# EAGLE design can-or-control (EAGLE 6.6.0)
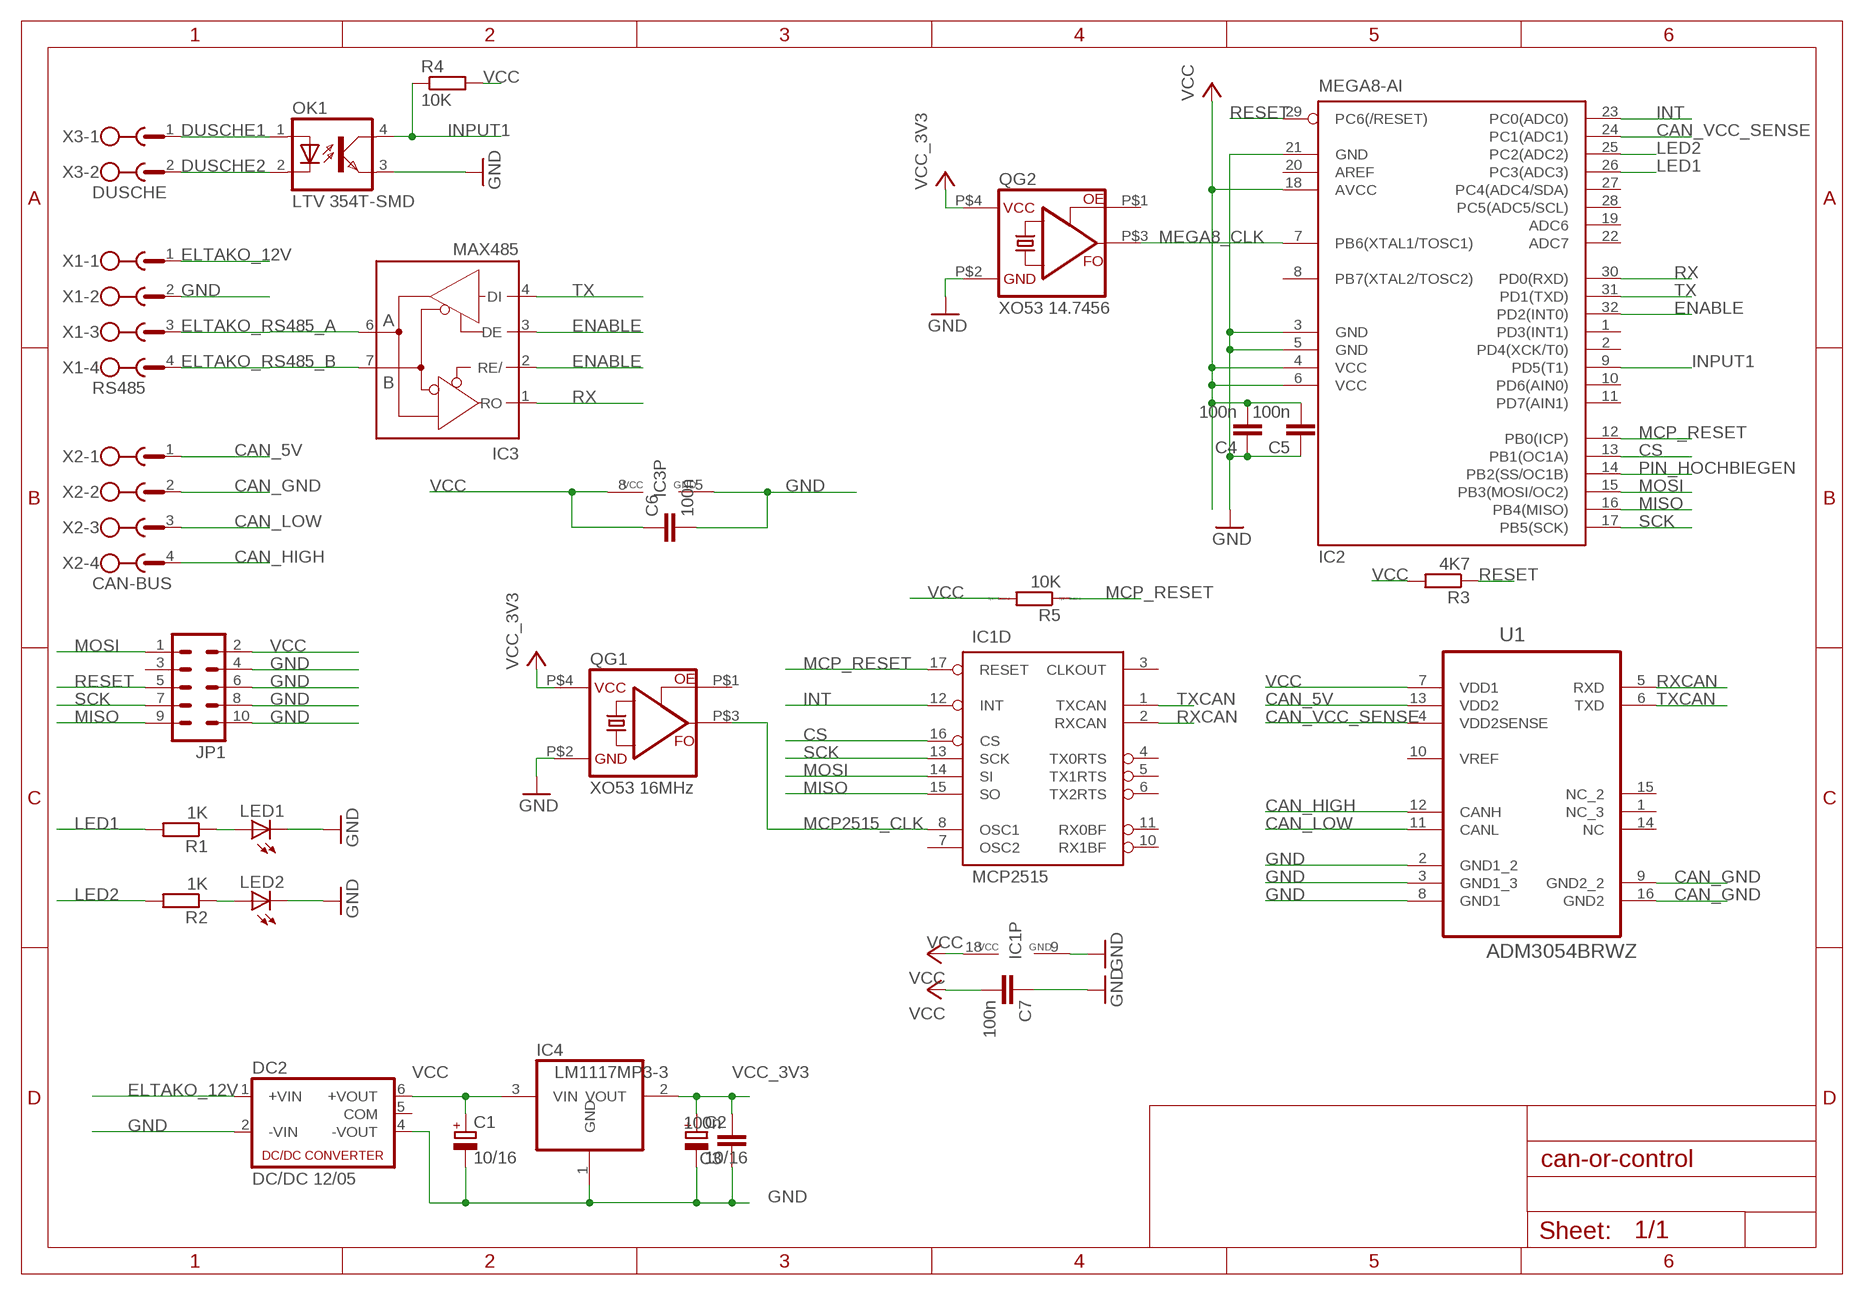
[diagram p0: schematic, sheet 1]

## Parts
C1  10/16  CPOL-EUSMCA  [SMC_A]
C2  10/16  CPOL-EUSMCA  [SMC_A]
C3  100n  C-EUC0805  [C0805]
C4  100n  C-EUC0805  [C0805]
C5  100n  C-EUC0805  [C0805]
C6  100n  C-EUC0805  [C0805]
C7  100n  C-EUC0805  [C0805]
DC2  DC/DC 12/05  NMA  [NMA]
IC1  MCP2515  MCP2515SO  [SO-18W]
IC2  MEGA8-AI  [TQFP32-08]
IC3  MAX485  MAX481CSA  [SO08]
IC4  LM1117MP3-3  REG1117  [SOT223]
JP1  ML10  [ML10]
LED1  LED3MM  [LED3MM]
LED2  LED3MM  [LED3MM]
OK1  LTV 354T-SMD  LTV816S  [SMD4]
QG1  XO53 16MHz  CRYSTALRESONATORXO53  [XO53]
QG2  XO53 14.7456  CRYSTALRESONATORXO53  [XO53]
R1  1K  R-EU_R0805  [R0805]
R2  1K  R-EU_R0805  [R0805]
R3  4K7  R-EU_R0805  [R0805]
R4  10K  R-EU_R0805  [R0805]
R5  10K  RR0603  [R0603]
U1  ADM3054BRWZ  [SOIC127P1032X265-16N]
X1  RS485  MSTBV4  [MSTBV4]
X2  CAN-BUS  MSTBV4  [MSTBV4]
X3  DUSCHE  MSTBV2  [MSTBV2]

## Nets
CAN_5V: U1.13(VDD2) X2.1
CAN_GND: U1.9(GND2_2) U1.16(GND2) X2.2
CAN_HIGH: U1.12(CANH) X2.4
CAN_LOW: U1.11(CANL) X2.3
CAN_VCC_SENSE: IC2.24(PC1(ADC1)) U1.4(VDD2SENSE)
CS: IC1.16(D:CS) IC2.13(PB1(OC1A))
DUSCHE1: OK1.1(A) X3.1
DUSCHE2: OK1.2(C) X3.2
ELTAKO_12V: DC2.1(+VIN) X1.1
ELTAKO_RS485_A: IC3.6(A) X1.3
ELTAKO_RS485_B: IC3.7(B) X1.4
ENABLE: IC2.32(PD2(INT0)) IC3.2(RE/) IC3.3(DE)
GND: C1.- C2.- C3.1 C4.1 C5.1 C6.2 C7.1 DC2.2(-VIN) DC2.4(-VOUT) IC1.9(P:GND) IC2.3(GND) IC2.5(GND) IC2.21(GND) IC3.5(GND) IC4.1(GND) JP1.4 JP1.6 JP1.8 JP1.10 LED1.K(C) LED2.K(C) OK1.3(EMIT) QG1.P$2(GND) QG2.P$2(GND) U1.2(GND1_2) U1.3(GND1_3) U1.8(GND1) X1.2
INPUT1: IC2.9(PD5(T1)) OK1.4(COL) R4.1
INT: IC1.12(D:INT) IC2.23(PC0(ADC0))
LED1: IC2.26(PC3(ADC3)) R1.2
LED2: IC2.25(PC2(ADC2)) R2.2
MCP2515_CLK: IC1.8(D:OSC1) QG1.P$3(FO)
MCP_RESET: IC1.17(D:RESET) IC2.12(PB0(ICP)) R5.1
MEGA8_CLK: IC2.7(PB6(XTAL1/TOSC1)) QG2.P$3(FO)
MISO: IC1.15(D:SO) IC2.16(PB4(MISO)) JP1.9
MOSI: IC1.14(D:SI) IC2.15(PB3(MOSI/OC2)) JP1.1
N$5: LED1.A R1.1
N$7: LED2.A R2.1
PIN_HOCHBIEGEN: IC2.14(PB2(SS/OC1B))
RESET: IC2.29(PC6(/RESET)) JP1.5 R3.1
RX: IC2.30(PD0(RXD)) IC3.1(RO)
RXCAN: IC1.2(D:RXCAN) U1.5(RXD)
SCK: IC1.13(D:SCK) IC2.17(PB5(SCK)) JP1.7
TX: IC2.31(PD1(TXD)) IC3.4(DI)
TXCAN: IC1.1(D:TXCAN) U1.6(TXD)
VCC: C1.+ C4.2 C5.2 C6.1 C7.2 DC2.6(+VOUT) IC1.18(P:VCC) IC2.4(VCC) IC2.6(VCC) IC2.18(AVCC) IC3.8(VCC) IC4.3(VIN) JP1.2 R3.2 R4.2 R5.2 U1.7(VDD1)
VCC_3V3: C2.+ C3.2 IC4.2(VOUT) QG1.P$4(VCC) QG2.P$4(VCC)
Unconnected: DC2.5(COM) IC1.3(D:CLKOUT) IC1.4(D:TX0RTS) IC1.5(D:TX1RTS) IC1.6(D:TX2RTS) IC1.7(D:OSC2) IC1.10(D:RX1BF) IC1.11(D:RX0BF) IC2.1(PD3(INT1)) IC2.2(PD4(XCK/T0)) IC2.8(PB7(XTAL2/TOSC2)) IC2.10(PD6(AIN0)) IC2.11(PD7(AIN1)) IC2.19(ADC6) IC2.20(AREF) IC2.22(ADC7) IC2.27(PC4(ADC4/SDA)) IC2.28(PC5(ADC5/SCL)) JP1.3 QG1.P$1(OE) QG2.P$1(OE) U1.1(NC_3) U1.10(VREF) U1.14(NC) U1.15(NC_2)

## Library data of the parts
C1 C2 = rcl:CPOL-EU: POLARIZED CAPACITOR, European symbol
C3-C7 = rcl:C-EU: CAPACITOR, European symbol
DC2 = dc-dc-converter:NMA: DC-DC CONVERTER; MF: C & D TECHNOLOGIES, INC; MPN: NMA0515SC; OC_FARNELL: 1021434; OC_NEWARK: 61K3064
IC1 = can:MCP2515: MC2515 Stand-Alone CAN Controller With SPI Interface, Microchip
IC2 = atmel:MEGA8: MICROCONTROLLER 8 Kbytes FLASH, 1 kbytes SRAM, 512 bytes EEPROM, USART, 6-channel 10 bit ADC, 2-channel 8 bit ADC Pin compatible with Atmega48, ATMega88, ATMega168 Source: avr.lbr; MPN: ATMEGA8-16AU; OC_FARNELL: 9171371; OC_NEWARK: 73M8863
IC3 = maxim:MAX481CSA: RS485 TRANSEIVER; MF: MAXIM; MPN: MAX481CSA; OC_FARNELL: unknown; OC_NEWARK: 90C3817
IC4 = burr-brown:REG1117: 800mA and 1A Low Dropout (LDO) Positive Regulator 1.8V, 2.5V, 2.85V, 3.3V, 5V, and Adj; MPN: REG1117; OC_FARNELL: 1097566; OC_NEWARK: 14P6981
JP1 = con-harting-ml:ML10: HARTING; OC_FARNELL: unknown; OC_NEWARK: unknown
LED1 LED2 = led:LED: LED
OK1 = optocoupler:LTV816: OPTO COUPLER Source: LITEON, LTV816.pdf; OC_FARNELL: unknown; OC_NEWARK: unknown
QG1 QG2 = Crystals-new:CRYSTALRESONATOR
R1-R4 = rcl:R-EU_: RESISTOR, European symbol
R5 = eagle-ltspice:R: RESISTOR, European symbol; SPICEMODEL: NONE; SPICEPREFIX: R
U1 = ADI-Phase-2:ADM3054BRWZ: 5kVrms Int Signal + Power ISO CAN Xcvr; MPN: ADM3054BRWZ; OC_FARNELL: 2095421; OC_NEWARK: 72T3514; PACKAGE: 16-Lead SOIC_W; SUPPLIER: Analog Devices
X1 X2 = con-phoenix-508:MSTBV4: PHOENIX; MPN: MSTBV 2,5/4-GF-5.08; OC_FARNELL: 1792794; OC_NEWARK: 69R9847
X3 = con-phoenix-508:MSTBV2: PHOENIX; MPN: MSTBV 2,5/2-GF-5.08; OC_FARNELL: 1792792; OC_NEWARK: 69R9845

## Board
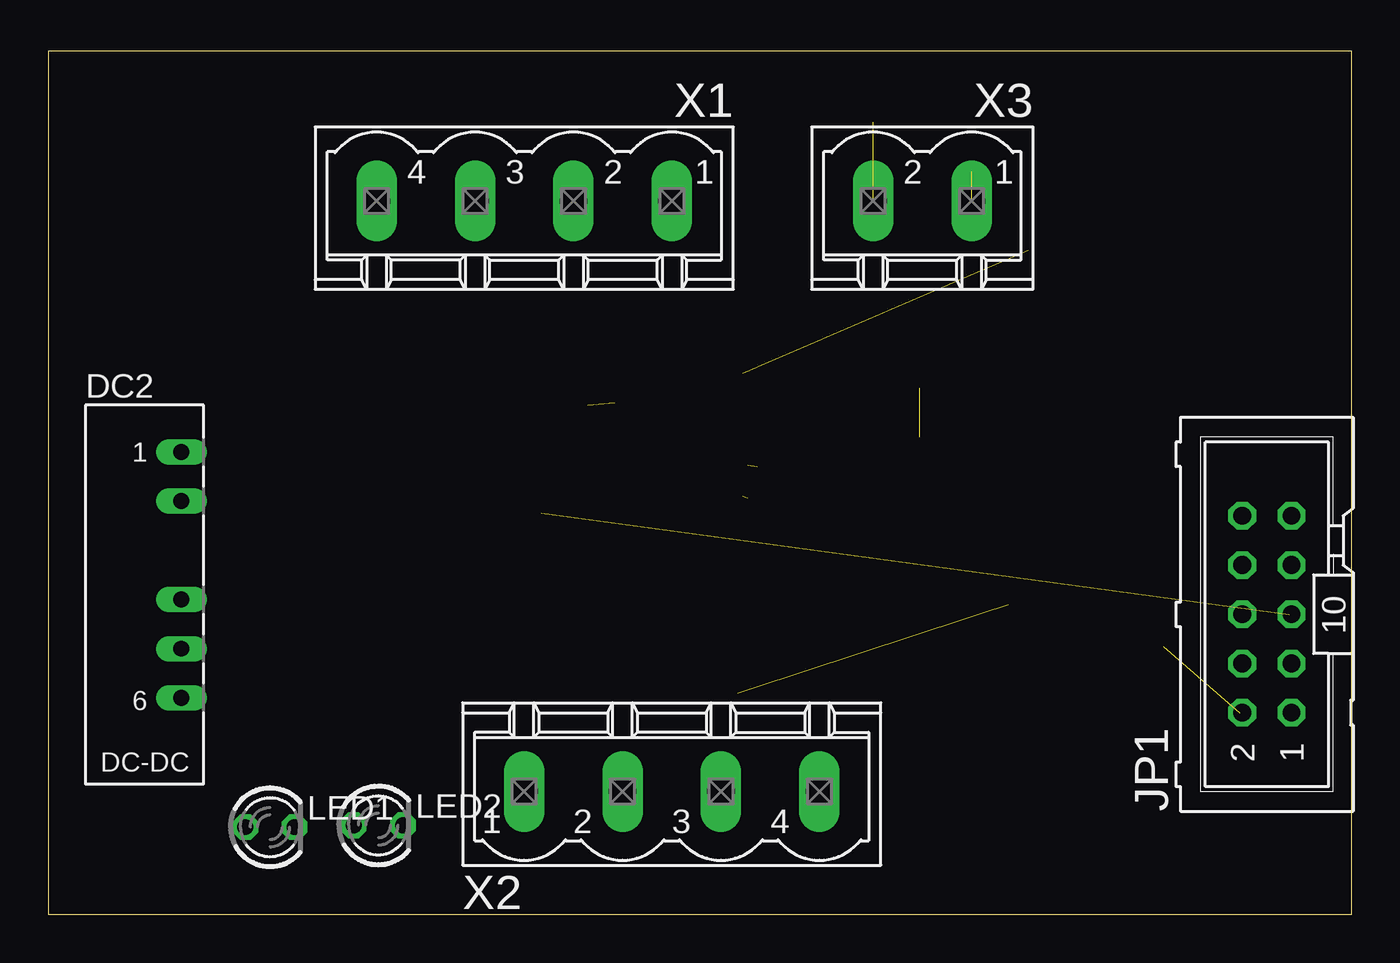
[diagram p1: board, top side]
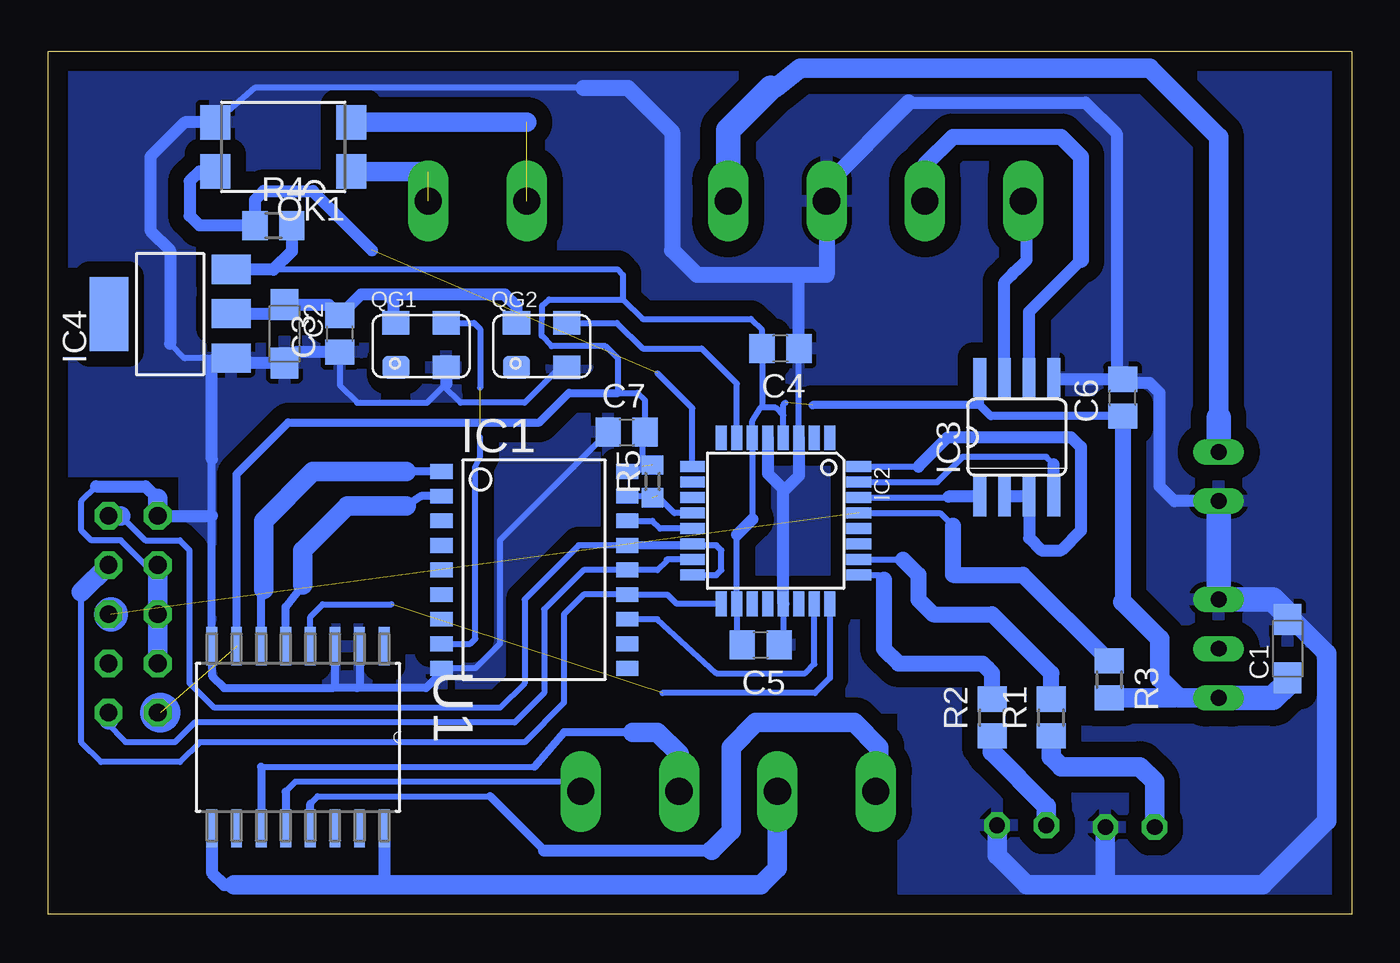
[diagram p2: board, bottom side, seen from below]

Size 67.23 x 44.57 mm. Coordinates in mm from the lower left corner, seen from the top.
Outline: 0,0 67.23,0 67.23,44.57 0,44.57 0,0
Copper layers (1*16): Top 0.035mm / dielectric 1.5mm / Bottom 0.035mm
Design rules "default": minimum track width 10mil, minimum drill 24mil, track to track 8mil, track to pad 8mil, pad to pad 8mil, via to via 8mil, smd to smd 8mil, copper to edge 40mil, drill to drill 8mil, minimum pad ring 10mil, minimum via ring 8mil, stop-mask expansion 4mil, vias tented up to drill 0mil, thermal gap 10mil
bRestrict: area 47,1.3 to 49.5,8.9

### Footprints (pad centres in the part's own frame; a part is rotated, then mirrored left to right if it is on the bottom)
SMC_A = smd 1.6 x 1.4: + -1.5,0; - 1.5,0
C0805 = smd 1.3 x 1.5: 1 -0.95,0; 2 0.95,0
NMA = drill 0.813 long: 1 0,6.35; 2 0,3.81; 4 0,-1.27; 5 0,-3.81; 6 0,-6.35
SO-18W = smd 0.762 x 1.143: 1 -5.08,-4.788; 2 -3.81,-4.788; 3 -2.54,-4.788; 4 -1.27,-4.788; 5 0,-4.788; 6 1.27,-4.788; 7 2.54,-4.788; 8 3.81,-4.788; 9 5.08,-4.788; 10 5.08,4.788; 11 3.81,4.788; 12 2.54,4.788; 13 1.27,4.788; 14 0,4.788; 15 -1.27,4.788; 16 -2.54,4.788; 17 -3.81,4.788; 18 -5.08,4.788
TQFP32-08 = smd 1.27 x 0.559: 1 -4.293,2.8; 2 -4.293,2; 3 -4.293,1.2; 4 -4.293,0.4; 5 -4.293,-0.4; 6 -4.293,-1.2; 7 -4.293,-2; 8 -4.293,-2.8; 17 4.293,-2.8; 18 4.293,-2; 19 4.293,-1.2; 20 4.293,-0.4; 21 4.293,0.4; 22 4.293,1.2; 23 4.293,2; 24 4.293,2.8 | smd 0.559 x 1.27: 9 -2.8,-4.293; 10 -2,-4.293; 11 -1.2,-4.293; 12 -0.4,-4.293; 13 0.4,-4.293; 14 1.2,-4.293; 15 2,-4.293; 16 2.8,-4.293; 25 2.8,4.293; 26 2,4.293; 27 1.2,4.293; 28 0.4,4.293; 29 -0.4,4.293; 30 -1.2,4.293; 31 -2,4.293; 32 -2.8,4.293
SO08 = smd 0.66 x 2.032: 1 -1.905,-3.073; 2 -0.635,-3.073; 3 0.635,-3.073; 4 1.905,-3.073; 5 1.905,3.073; 6 0.635,3.073; 7 -0.635,3.073; 8 -1.905,3.073
SOT223 = smd 1.499 x 2.007: 1 -2.261,-3.15; 2 0.025,-3.15; 3 2.311,-3.15 | smd 3.81 x 2.007: 4 0,3.15
ML10 = drill 0.914 octagon: 1 -5.08,-1.27; 2 -5.08,1.27; 3 -2.54,-1.27; 4 -2.54,1.27; 5 0,-1.27; 6 0,1.27; 7 2.54,-1.27; 8 2.54,1.27; 9 5.08,-1.27; 10 5.08,1.27
LED3MM = drill 0.813 octagon: A -1.27,0; K 1.27,0
SMD4 = smd 1.78 x 1.55: 1 -1.27,-3.5; 2 1.27,-3.5; 3 1.27,3.5; 4 -1.27,3.5
XO53 = smd 1.4 x 1.2: P$1 -1.3,-1.1; P$2 1.3,-1.1; P$3 1.3,1.2; P$4 -1.3,1.2
R0805 = smd 1.3 x 1.5: 1 -0.95,0; 2 0.95,0
R0603 = smd 1 x 1.1: 1 -0.85,0; 2 0.85,0
SOIC127P1032X265-16N = smd 1.981 x 0.559: 1 -4.699,4.445; 2 -4.699,3.175; 3 -4.699,1.905; 4 -4.699,0.635; 5 -4.699,-0.635; 6 -4.699,-1.905; 7 -4.699,-3.175; 8 -4.699,-4.445; 9 4.699,-4.445; 10 4.699,-3.175; 11 4.699,-1.905; 12 4.699,-0.635; 13 4.699,0.635; 14 4.699,1.905; 15 4.699,3.175; 16 4.699,4.445
MSTBV4 = drill 1.397 long: 1 -7.62,0; 2 -2.54,0; 3 2.54,0; 4 7.62,0
MSTBV2 = drill 1.397 long: 1 -2.54,0; 2 2.54,0

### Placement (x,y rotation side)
C1  3.3,13.72 90 bottom
C2  55.05,29.97 270 bottom
C3  52.2,29.97 90 bottom
C4  29.46,29.21 180 bottom
C5  30.48,13.91 180 bottom
C6  11.81,26.67 90 bottom
C7  37.4,24.89 0 bottom
DC2  6.86,17.53 0 top
IC1  42.16,17.78 270 bottom
IC2  29.72,20.32 270 bottom
IC3  17.27,24.64 0 bottom
IC4  60.96,30.99 90 bottom
JP1  62.87,15.49 90 top
LED1  11.43,4.51 0 top
LED2  17.02,4.6 0 top
OK1  55.12,39.62 90 bottom
QG1  48.01,29.34 0 bottom
QG2  41.78,29.34 0 bottom
R1  15.49,10.16 90 bottom
R2  18.54,10.16 90 bottom
R3  12.51,12.13 270 bottom
R4  55.63,35.56 0 bottom
R5  36.07,22.35 90 bottom
U1  54.36,9.14 270 bottom
X1  24.55,36.83 180 top
X2  32.16,6.35 0 top
X3  45.09,36.83 180 top

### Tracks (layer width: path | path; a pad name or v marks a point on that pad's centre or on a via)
CAN_5V
  Bottom 0.305: 53.72,5.71 53.34,6.1 44.45,6.1
  Bottom 0.406: U1.13 53.72,5.71 | 44.45,6.1 41.66,3.3
  Bottom 0.61: 41.66,3.3 33.02,3.3
  Bottom 1.016: 33.02,3.3 32,4.32 32,8.64 30.73,9.91 25.65,9.91 24.38,8.64 24.38,6.51 X2.1
CAN_GND
  Bottom 0.61: U1.9 58.8,2.16 58.17,1.52 57.66,1.52 | U1.16 49.91,1.91 49.53,1.52
  Bottom 1.016: X2.2 29.62,2.38 30.48,1.52 49.53,1.52 57.66,1.52
CAN_HIGH
  Bottom 0.305: 54.99,6.35 54.48,6.86 39.62,6.86
  Bottom 0.406: 54.99,6.35 U1.12 | 39.62,6.86 39.78,6.7 X2.4
CAN_LOW
  Bottom 0.305: 56.26,7.62 42.16,7.62
  Bottom 0.406: 37.08,9.4 40.64,9.4 42.16,7.62 | 56.26,7.62 U1.11
  Bottom 1.016: 37.08,9.4 35.81,9.4 34.7,8.28 X2.3
CAN_VCC_SENSE  (1 unrouted)
  Bottom 0.305: U1.4 53.72,15.37 53.09,16 49.53,16 | IC2.24 26.92,12.2 27.69,11.43 35.56,11.43
CS
  Bottom 0.305: IC1.16 36.07,20.32 35.67,19.92 IC2.13
DUSCHE1  (1 unrouted)
  Bottom 1.016: OK1.1 47.63,38.35
DUSCHE2  (1 unrouted)
  Bottom 1.016: OK1.2 42.55,40.89
ELTAKO_12V
  Bottom 0.406: 29.97,42.67 29.72,42.67
  Bottom 1.016: 29.72,42.67 28.45,43.69 10.41,43.69 6.86,40.13 6.86,25.65
  Bottom 1.27: DC2.1 6.86,25.65 | 29.97,42.67 32.17,40.47 X1.1
ELTAKO_RS485_A
  Bottom 0.61: 13.97,33.78 16.64,31.11 IC3.6
  Bottom 0.813: X1.3 22.01,38.7 20.57,40.13 14.99,40.13 13.97,39.12 13.97,33.78
ELTAKO_RS485_B
  Bottom 0.61: X1.4 16.76,36.66 16.76,33.78 17.14,33.4 17.53,33.02 17.91,32.64 IC3.7
ENABLE
  Bottom 0.305: IC2.32 22.35,23.12
  Bottom 0.61: IC3.2 IC3.3 16.64,19.43 16,18.8 14.99,18.8 13.97,19.81 13.97,24.13 14.48,24.64 20.83,24.64 22.35,23.12
GND
  Bottom 0.305: 29.32,21.84 29.32,21.95 | 46.95,12.48 IC1.9 45.21,12.7 43.94,13.97 43.94,19.3 40.13,23.12 C7.1 | JP1.8 62.23,18.03 63.5,19.3 65.02,19.3 65.53,19.81 65.53,21.34 64.77,22.1 | C1.- 3.3,15.49 | IC2.21 29.32,14.12 C5.1 | 54.51,29.02 C2.- | 57.55,28.47 IC4.1 58.67,28.73 | 60.96,29.46 60.2,28.7 60.17,28.73 58.67,28.73 | 39.62,42.67 56.59,42.67 OK1.3 | 58.8,28.6 58.67,28.73 | 46.83,27.27 45.97,26.42 42.67,26.42 41.12,27.97 40.75,27.97 QG2.P$2 | C3.1 52.2,27.3 51.31,26.42 47.69,26.42 46.83,27.27 | IC2.3 C4.1 | 46.71,27.4 46.83,27.27
  Bottom 0.406: 58.8,23.5 58.8,20.57 U1.8 58.8,12.32 58.17,11.68 52.58,11.68 | U1.3 52.45,11.81 52.58,11.68 | 46.95,12.48 47.75,11.68 51.31,11.68 | 51.31,11.68 52.58,11.68 | U1.2 51.18,11.81 51.31,11.68 | 15.37,28.32 IC3.5 15.28,27.62 | 12.13,27.93 C6.2 11.62,27.43
  Bottom 0.61: 22.86,41.91 13.72,41.91 12.13,40.32 12.13,27.93 | IC2.21 29.32,21.84 28.52,22.64 IC2.3 | 29.32,21.95 30.12,22.75 IC2.5 | 64.77,22.1 62.23,22.1 61.59,21.46 | JP1.10 58.8,20.57 | C3.1 54.51,29.02 | C2.- 57.55,28.47 | OK1.3 60.2,40.89 61.98,39.12 61.98,35.31 60.96,34.29 60.96,29.46 | 58.8,23.5 58.8,28.6 | DC2.2 9.14,21.34 9.91,22.1 9.91,26.92 10.41,27.43 11.62,27.43 | C6.2 15.28,27.62 | C4.1 28.51,33.02 28.45,33.02 | QG1.P$2 46.71,27.4
  Bottom 0.813: 22.86,41.91 27.09,37.68 X1.2 27.09,33.02 28.45,33.02 33.78,33.02 35.05,34.29 35.05,40.39 37.34,42.67 39.62,42.67
  Bottom 1.016: JP1.8 JP1.6 JP1.4 | JP1.10 61.59,21.46 | LED2.K 18.29,3.05 16.76,1.52 12.7,1.52 | 12.7,1.52 4.57,1.52 1.27,4.83 1.27,13.46 3.68,15.88 | LED1.K 12.7,1.52
  Bottom 1.27: DC2.2 DC2.4 4.06,16.26 3.68,15.88 3.3,15.49
  pour Bottom (isolate 0.813, rank 3): 0,0 23.11,0 23.11,10.67 60.2,10.67 60.2,22.86 67.31,22.86 67.31,44.45 0,44.45
INPUT1  (1 unrouted)
  Bottom 0.305: OK1.4 59.44,38.35 | IC2.9 34.01,26.14 35.81,27.94
  Bottom 0.61: 59.44,38.35 59.94,37.85 59.94,36.07 59.44,35.56 R4.1 56.58,36.9 56.13,37.34 53.59,37.34 50.55,34.29
INT
  Bottom 0.305: IC1.12 35.81,15.24 32.77,12.45 28.19,12.45 27.72,12.92 IC2.23
LED1
  Bottom 0.305: IC2.26 23.15,18.32
  Bottom 0.813: 23.15,18.32 22.35,17.53 22.35,16.26 21.59,15.49 18.54,15.49 15.49,12.45 R1.2
LED2
  Bottom 0.305: IC2.25 24.38,17.52 24.13,17.27
  Bottom 0.813: R2.2 18.54,12.45 18.8,12.7 19.05,12.95 23.37,12.95 24.13,13.72 24.13,17.27
MCP2515_CLK  (1 unrouted)
  Bottom 0.305: IC1.8 45.47,13.97 45.21,14.22 45.21,23.11 44.96,23.62 44.96,24.64 | QG1.P$3 45.27,30.54 44.96,30.23 44.96,27.18
MCP_RESET  (1 unrouted)
  Bottom 0.305: IC2.12 34.94,20.72 35.81,21.59 IC1.17
MEGA8_CLK
  Bottom 0.305: QG2.P$3 37.9,30.54 36.58,29.21 33.53,29.21 31.72,27.4 IC2.7
MISO
  Bottom 0.305: IC2.16 32.77,17.52 32.51,17.78 32.51,18.8 32.77,19.05 33.94,19.05 | 37.31,19.12 IC1.15 | IC1.15 37.34,19.05 | IC1.15 39.88,19.05 42.67,16.26 42.67,11.94 43.94,10.67 58.67,10.67 59.94,11.94 59.94,18.8 60.45,19.3 62.23,19.3 63.5,20.57
  Bottom 0.406: 33.94,19.05 IC1.15
  Bottom 1.016: JP1.9 63.5,20.57
MOSI
  Bottom 0.305: IC2.15 35.34,18.32 35.34,18.26 35.81,17.78 IC1.14 39.62,17.78 41.66,15.75 41.66,11.43 43.18,9.91 59.69,9.91 60.71,8.89 63.25,8.89 64.26,9.91 64.14,10.03
  Bottom 1.016: JP1.1 64.14,10.03
N$5
  Bottom 1.016: LED1.A 10.16,6.86 10.92,7.62 14.99,7.62 15.49,8.13 R1.1
N$7
  Bottom 1.016: LED2.A 15.75,5.59 18.54,8.38 R2.1
RESET  (1 unrouted)
  Bottom 0.305: IC2.29 21.23,20.72 20.57,20.07
  Bottom 0.813: 20.57,20.07 20.57,17.53 16.96,17.53 R3.1 | JP1.5 64.01,15.49
RX
  Bottom 0.305: IC2.30 20.85,21.52 20.8,21.57
  Bottom 0.61: IC3.1 20.8,21.57
RXCAN
  Bottom 0.406: IC1.2 48.01,21.59 48.77,21.08 | U1.5 54.99,15.88 54.1,17.02
  Bottom 1.016: 54.1,17.02 54.1,18.8 51.82,21.08 48.77,21.08
SCK
  Bottom 0.305: IC2.17 34.82,16.03 35.31,16.51 IC1.13 39.62,16.51 40.64,15.49 40.64,10.92 42.67,8.89 59.44,8.89 60.45,7.87 64.52,7.87 65.53,8.89 65.53,16.64
  Bottom 1.016: 65.53,16.64 JP1.7
TX
  Bottom 0.305: 15.37,23.24 15.75,23.62 20.07,23.62 21.37,22.32 IC2.31
  Bottom 0.61: IC3.4 15.37,23.24
TXCAN
  Bottom 0.406: IC1.1 48.77,22.86 | U1.6 56.26,16.64 56.13,16.76
  Bottom 1.016: 48.77,22.86 53.59,22.86 56.13,20.32 56.13,16.76
VCC  (3 unrouted)
  Bottom 0.305: 30.92,20.39 IC2.6 30.92,25.47 30.48,26.16 | 31.72,19.59 IC2.18 31.72,14.19 C5.2 31.43,14.16 31.5,14.22 | IC2.4 29.32,25.76 | 30.48,26.16 29.72,26.16 29.32,25.76 | C1.+ 3.3,11.94 | 57.78,33.27 IC4.3 37.87,33.3 37.59,33.02 37.59,31.75 | IC1.18 36.83,22.86 36.58,23.11 36.58,24.77 C7.2 36.45,26.55 36.83,26.92 37.85,26.92 37.85,28.7 38.48,29.34 41.27,29.34 41.78,29.87 41.76,31.42 41.4,31.75 37.59,31.75 | 29.32,25.76 29.32,26.31 29.21,26.42 | 30.48,26.16 30.41,26.23 C4.2 30.41,30.16 30.99,30.73 36.58,30.73 37.59,31.75
  Bottom 0.406: U1.7 57.53,22.73 54.86,25.4 41.91,25.4 40.39,26.92 37.85,26.92 | C6.1 18.61,25.72 19.18,26.29 | IC3.8 19.18,26.29 | 8.89,11.18 9.02,11.3 9.14,11.18 | 19.18,26.29 27.81,26.29
  Bottom 0.61: 30.92,20.39 31.72,19.59 | R4.2 54.68,34.22 55.63,33.27 57.78,33.27
  Bottom 0.813: C6.1 11.81,16.13 | JP1.2 61.47,10.41
  Bottom 1.016: 11.81,16.13 9.91,14.22 9.91,12.19 9.02,11.3 | 8.89,11.18 DC2.6 | R3.2 9.14,11.18
  Bottom 1.27: 3.3,11.94 4.06,11.18 DC2.6
VCC_3V3
  Bottom 0.305: 55.51,31.01 C2.+ | 52.75,31.47 C3.2 | 49.43,30.66 QG1.P$4
  Bottom 0.61: IC4.2 55.51,31.01 | C2.+ 52.75,31.47 | C3.2 51.12,32 49.78,32 | 49.78,32 43.69,32 43.08,31.4 QG2.P$4 | 49.78,32 49.43,31.65 49.43,30.66
(copper drawn outside any net)
  shapes: Bottom circle x2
